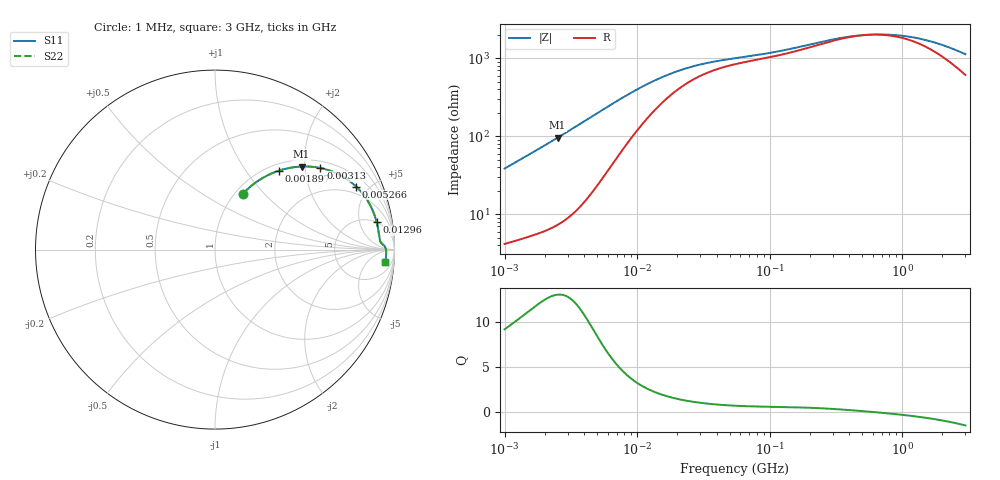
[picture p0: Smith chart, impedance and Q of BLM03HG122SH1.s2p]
! BLM03HG122SH1
# Hz S RI R 50
!Freq.(Hz) S11(Real) S11(Imag) S21(Real) S21(Imag) S12(Real) S12(Imag) S22(Real) S22(Imag)
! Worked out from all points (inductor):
!   401 points, 1 MHz to 3 GHz, reference 50 ohm
!   read as one part in series: L = 6.09 uH near 1.041 MHz
!   highest Q = 13.1 at 2.511 MHz (marker M1), where L = 6.08 uH
!   self-resonance near 552.2 MHz
!   S11 on the Smith chart (normalised r, x): 1 MHz: 1.08, +0.77; 1.897 MHz: 1.12, +1.45; 3.13 MHz: 1.19, +2.41; 5.266 MHz: 1.53, +4.16; 12.96 MHz: 5, +9; 3 GHz: 13, -19
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1000000  0.1555 0.312  0.8445 -0.312  0.8445 -0.312  0.1555 0.312
1377479  0.2385 0.3821  0.7615 -0.3821  0.7615 -0.3821  0.2385 0.3821
1897447  0.3558 0.4397  0.6442 -0.4397  0.6442 -0.4397  0.3558 0.4397
2511129  0.4823 0.4629  0.5177 -0.4629  0.5177 -0.4629  0.4823 0.4629
3129607  0.5869 0.4544  0.4131 -0.4544  0.4131 -0.4544  0.5869 0.4544
3823119  0.6757 0.4257  0.3243 -0.4257  0.3243 -0.4257  0.6757 0.4257
5266264  0.7866 0.351  0.2134 -0.351  0.2134 -0.351  0.7866 0.351
7858845  0.8641 0.2486  0.1359 -0.2486  0.1359 -0.2486  0.8641 0.2486
1.29622e7  0.9007 0.1526  0.0993 -0.1526  0.0993 -0.1526  0.9007 0.1526
1.461624e7  0.9047 0.1357  0.0953 -0.1357  0.0953 -0.1357  0.9047 0.1357
1.973457e7  0.911 0.102  0.089 -0.102  0.089 -0.102  0.911 0.102
2.664524e7  0.9146 0.078  0.0854 -0.078  0.0854 -0.078  0.9146 0.078
5.477226e7  0.9207 0.0462  0.0793 -0.0462  0.0793 -0.0462  0.9207 0.0462
1.103592e8  0.9306 0.0332  0.0694 -0.0332  0.0694 -0.0332  0.9306 0.0332
2.094008e8  0.9426 0.0222  0.0574 -0.0222  0.0574 -0.0222  0.9426 0.0222
4.304467e8  0.9511 0.00601  0.0489 -0.00601  0.0489 -0.00601  0.9511 0.00601
5.929311e8  0.9528 -0.00176  0.0472 0.00176  0.0472 0.00176  0.9528 -0.00176
8.005644e8  0.9536 -0.00959  0.0464 0.00959  0.0464 0.00959  0.9536 -0.00959
1.10276e9  0.9538 -0.0191  0.0462 0.0191  0.0462 0.0191  0.9538 -0.0191
1.519029e9  0.9535 -0.0306  0.0465 0.0306  0.0465 0.0306  0.9535 -0.0306
2.050964e9  0.9524 -0.0442  0.0476 0.0442  0.0476 0.0442  0.9524 -0.0442
3e9  0.9496 -0.0673  0.0504 0.0673  0.0504 0.0673  0.9496 -0.0673
